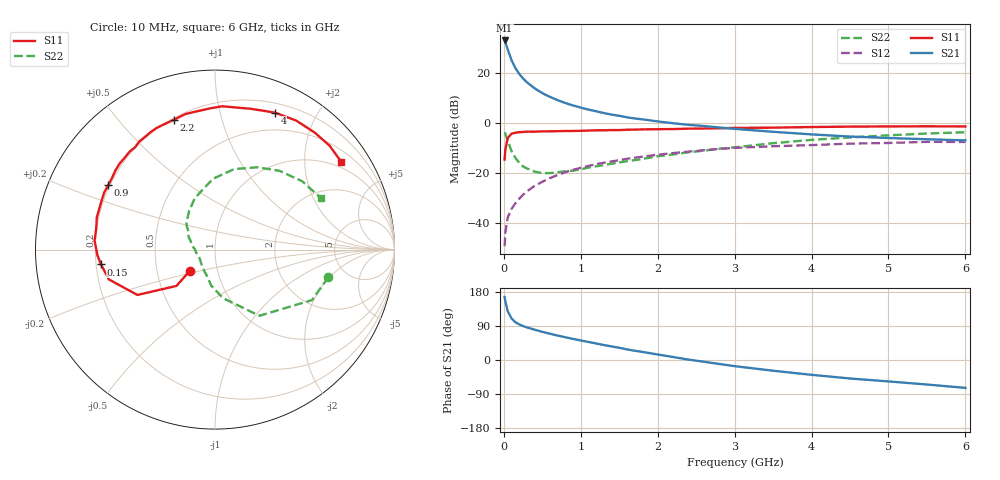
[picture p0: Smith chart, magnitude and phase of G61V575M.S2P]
! SIEMENS Small Signal Semiconductors
! BFG193
! Si NPN RF Bipolar Junction Transistor in SOT223
! VCE = 1.5 V  IC = 75 mA
! Common Emitter S-Parameters:  August  1996
# GHz  S  MA  R  50
!  f  S11  S21  S12  S22
! GHz  MAG  ANG  MAG  ANG  MAG  ANG  MAG  ANG
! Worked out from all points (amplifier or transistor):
!   36 points, 10 MHz to 6 GHz, reference 50 ohm
!   highest |S21| = 33.1 dB at 10 MHz (marker M1)
!   |S21| within 3 dB of that: start of sweep to 44.08 MHz
!   unconditionally stable (mu >= 1): start of sweep to 23.21 MHz; 141.5 MHz to end of sweep
!   at 250 MHz: K = 1.11, MAG = 21.3 dB, |S12| = -28.7 dB
!   at 1.4 GHz: K = 1.15, MAG = 7.0 dB, |S12| = -15.4 dB
!   at 6 GHz: K = 1.04, MAG = -0.9 dB, |S12| = -7.6 dB
!   S11 on the Smith chart (normalised r, x): 10 MHz: 0.73, -0.18; 150 MHz: 0.22, -0.06; 900 MHz: 0.19, +0.27; 2.2 GHz: 0.21, +0.71; 4 GHz: 0.30, +1.49; 6 GHz: 0.81, +2.99
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0.01  0.1856 -139.8  45.38 166.2  0.0034 71.9  0.6495 -13.8
0.02  0.2949 -136.7  42.05 154.2  0.0064 69.1  0.6091 -27.5
0.05  0.5008 -149.7  30.07 128.6  0.0127 60.7  0.4442 -56.1
0.1  0.6142 -164.3  18.29 109.8  0.019 60.8  0.2743 -80.6
0.15  0.6407 -172.6  12.68 99.8  0.0247 62.1  0.2012 -96.1
0.2  0.6558 -177.2  9.735 94.0  0.0304 65.3  0.16 -104.8
0.25  0.6637 178.9  7.835 89.5  0.0366 66.4  0.1349 -115.6
0.3  0.6729 175.8  6.586 86.0  0.0428 67.9  0.1232 -122.8
0.4  0.6719 170.1  4.974 80.0  0.0548 67.9  0.1067 -137.4
0.5  0.6824 164.8  3.991 74.4  0.0666 67.0  0.099 -148.8
0.6  0.6837 160.6  3.347 69.4  0.079 65.5  0.0991 -156.9
0.7  0.6882 156.6  2.88 64.5  0.0911 63.8  0.1033 -165.0
0.9  0.6946 148.9  2.255 55.6  0.1156 59.8  0.1111 -180.0
1.1  0.7085 141.6  1.865 47.6  0.1382 55.7  0.1281 171.0
1.6  0.7355 124.9  1.305 28.1  0.1924 43.7  0.172 150.3
2.2  0.759 107.4  0.993 7.9  0.2504 28.9  0.2342 130.7
2.8  0.7876 91.8  0.816 -10.5  0.3032 14.1  0.3053 112.0
3.5  0.8098 75.6  0.669 -28.3  0.3429 -4.1  0.3948 91.6
4  0.8331 66.3  0.593 -39.1  0.3616 -14.0  0.4607 76.7
4.5  0.8493 57.8  0.537 -48.8  0.387 -24.1  0.5154 62.9
5.5  0.8618 42.2  0.474 -64.7  0.4198 -47.0  0.6175 38.0
6  0.8568 34.8  0.45 -73.6  0.4181 -59.9  0.6556 26.1
